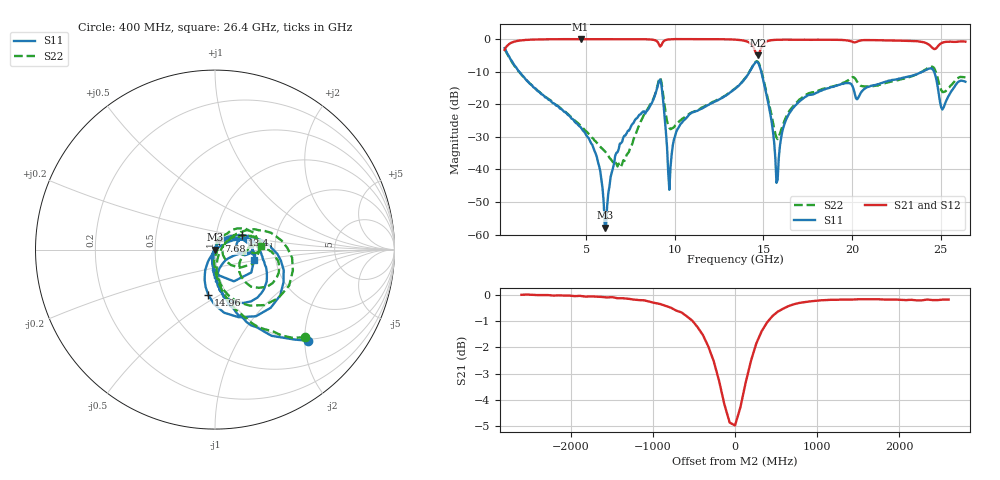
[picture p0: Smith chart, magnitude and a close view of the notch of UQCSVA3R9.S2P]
!  Part Number  UQCSVA3R9  Mounting Orientation: Horizontal
!  Description: Ultra Low ESR Microwave capacitors
!  Application: Coupling, Bypass, Tuning, DC Block
!  Filters, Matching
# GHZ S DB R 50
! Freq  |S11|  S11 Ph  |S21|  S21 Ph  |S12|  S12 Ph  |S22|  S22 Ph
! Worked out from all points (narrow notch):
!   401 points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, 400 MHz to 26.4 GHz, reference 50 ohm
!   highest |S21| = 0.00 dB at 4.69 GHz (marker M1); lowest = -5.0 dB at 14.7 GHz (marker M2)
!   notch at M2: 4.8 dB deep, 443 MHz wide at half that depth
!   lowest |S11| = -57.9 dB at 6.055 GHz (marker M3), VSWR 1.00, Z = 50 - j0.122 ohm
!   |S11| at or under -10 dB: 1.225 GHz to 14.23 GHz (13 GHz wide, 168 % of centre); 14.88 GHz to 23.98 GHz (9.095 GHz wide, 46.8 % of centre); 24.64 GHz to end of sweep
!   |S22| runs from -39.1 to -3.1 dB; largest |S21 - S12| = 0.024
!   S11 on the Smith chart (normalised r, x): 400 MHz: 0.97, -2.08; 7.68 GHz: 1.04, +0.10; 13.4 GHz: 1.34, +0.22; 14.96 GHz: 0.82, -0.45; 26.4 GHz: 1.53, -0.18
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0.4  -2.77 -44.3  -3.31 45.0  -3.53 45.5  -3.08 -44.1
1.505  -11.74 -80.4  -0.31 10.1  -0.36 11.0  -11.86 -77.8
4.69  -27.01 -102.7  0.00 -12.8  -0.01 -12.8  -26.53 -91.1
4.755  -27.51 -102.0  0.00 -13.1  -0.01 -13.1  -26.99 -90.5
5.665  -37.65 -106.5  -0.01 -17.6  -0.01 -17.7  -32.13 -73.8
6.055  -57.85 -71.7  -0.01 -19.6  -0.01 -19.6  -34.39 -59.9
6.77  -34.74 69.9  -0.01 -22.9  -0.01 -22.2  -39.07 -9.4
7.68  -25.66 65.7  -0.01 -27.4  -0.01 -27.4  -30.62 71.0
9.11  -12.91 -7.4  -1.60 -39.1  -1.56 -39.0  -12.43 22.4
9.305  -16.72 -81.0  -1.19 -25.1  -1.18 -25.6  -15.32 -36.3
9.695  -46.23 124.3  -0.09 -31.1  -0.08 -31.4  -27.22 -15.4
10.41  -25.64 59.5  -0.01 -36.5  -0.01 -36.8  -24.47 29.8
13.4  -15.27 27.5  -0.16 -53.8  -0.16 -54.0  -15.16 34.4
14.7  -7.21 -58.4  -4.97 -48.9  -4.90 -49.0  -7.04 -37.3
14.96  -11.79 -98.2  -1.85 -38.0  -1.85 -38.1  -11.34 -73.0
15.805  -43.20 4.7  -0.21 -52.3  -0.22 -52.4  -30.68 -21.7
16.325  -24.20 31.7  -0.18 -56.3  -0.19 -56.5  -23.46 32.0
17.755  -17.01 20.4  -0.22 -63.9  -0.22 -64.2  -16.33 28.6
22.11  -12.73 8.4  -0.44 -83.7  -0.44 -83.5  -13.19 5.9
24.45  -8.95 -48.5  -2.22 -100.2  -2.18 -100.0  -8.46 -19.9
25.1  -21.59 -47.1  -1.11 -88.5  -1.08 -88.5  -16.23 -27.9
26.4  -13.08 -14.6  -0.79 -102.2  -0.74 -101.9  -11.78 4.3
